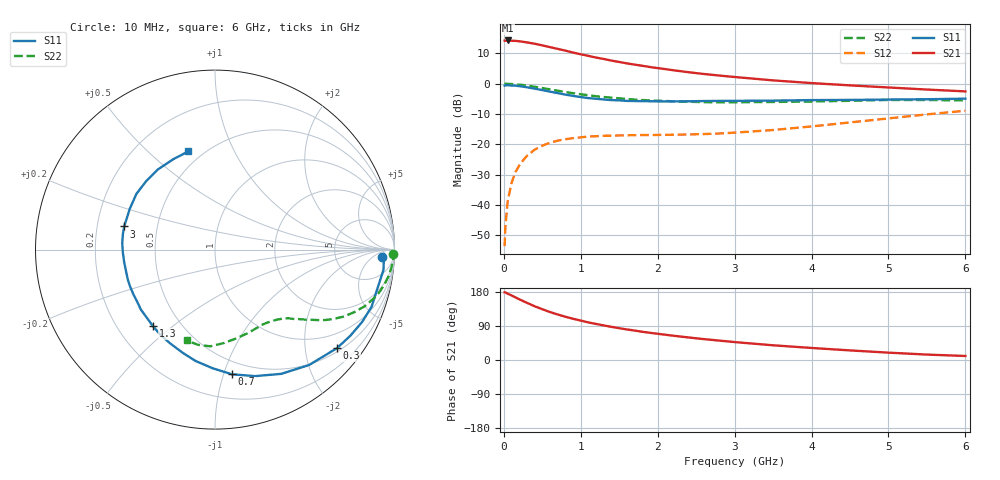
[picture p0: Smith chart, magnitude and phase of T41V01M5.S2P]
! Infineon Technologies  Discrete & RF Semiconductors
! BFR182T
! Si NPN RF Bipolar Junction Transistor in SC75
! VCE = 1 V  IC = 1.5 mA
! Common Emitter S-Parameters:  October  1999
# GHz  S  MA  R  50
!  f  S11  S21  S12  S22
! GHz  MAG  ANG  MAG  ANG  MAG  ANG  MAG  ANG
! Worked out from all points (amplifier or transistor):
!   36 points, 10 MHz to 6 GHz, reference 50 ohm
!   highest |S21| = 14.3 dB at 50 MHz (marker M1)
!   |S21| within 3 dB of that: start of sweep to 738.3 MHz
!   unconditionally stable (mu >= 1): 2.07 GHz to 4.762 GHz
!   at 250 MHz: K = 0.12, MSG = 19.5 dB, |S12| = -25.2 dB
!   at 1.4 GHz: K = 0.72, MSG = 12.4 dB, |S12| = -17.1 dB
!   at 6 GHz: K = 0.90, MSG = 3.2 dB, |S12| = -8.9 dB
!   S11 on the Smith chart (normalised r, x): 10 MHz: 21, -13; 300 MHz: 0.59, -2.72; 700 MHz: 0.39, -1.07; 1.3 GHz: 0.35, -0.43; 3 GHz: 0.32, +0.11; 6 GHz: 0.42, +0.68
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0.01  0.9334 -2.4  5.129 178.5  0.0021 86.9  0.9892 -1.3
0.02  0.9422 -1.4  5.112 178.4  0.0044 88.1  0.9999 -1.2
0.05  0.9455 -6.9  5.164 175.0  0.0116 87.0  0.9948 -2.9
0.1  0.9313 -12.9  5.106 170.4  0.0231 83.2  0.9879 -5.8
0.15  0.9287 -20.1  5.084 165.2  0.0347 78.5  0.9789 -8.6
0.2  0.9132 -26.3  5.005 160.3  0.0449 75.4  0.9654 -11.2
0.3  0.8739 -38.9  4.793 150.9  0.0648 68.3  0.9331 -16.3
0.4  0.8297 -50.8  4.562 141.8  0.0817 61.6  0.8911 -20.8
0.5  0.7846 -61.9  4.287 134.0  0.0951 56.4  0.8478 -24.4
0.6  0.7396 -72.4  4.008 126.5  0.1067 51.8  0.8069 -27.6
0.7  0.7009 -82.3  3.75 120.1  0.1151 47.9  0.7664 -30.2
0.9  0.6299 -99.9  3.265 108.8  0.1269 41.6  0.6972 -34.3
1.1  0.5791 -115.6  2.875 99.1  0.1346 37.6  0.6453 -37.3
1.3  0.5487 -129.1  2.555 91.2  0.1387 34.7  0.6034 -39.9
1.5  0.5313 -141.0  2.283 83.9  0.1404 33.4  0.5742 -42.1
1.8  0.5158 -156.5  1.975 74.5  0.1427 32.6  0.5377 -45.7
2.2  0.5108 -171.8  1.67 64.1  0.1443 34.4  0.5135 -50.3
3  0.5221 165.7  1.29 47.3  0.1562 41.9  0.4947 -61.0
3.5  0.5266 154.3  1.135 38.8  0.1725 47.2  0.5003 -68.9
4.5  0.5406 135.4  0.939 25.3  0.23 53.3  0.5231 -84.7
5.5  0.5547 114.8  0.801 14.3  0.3122 52.4  0.539 -100.1
6  0.567 105.1  0.747 10.6  0.3589 49.6  0.5302 -107.3
